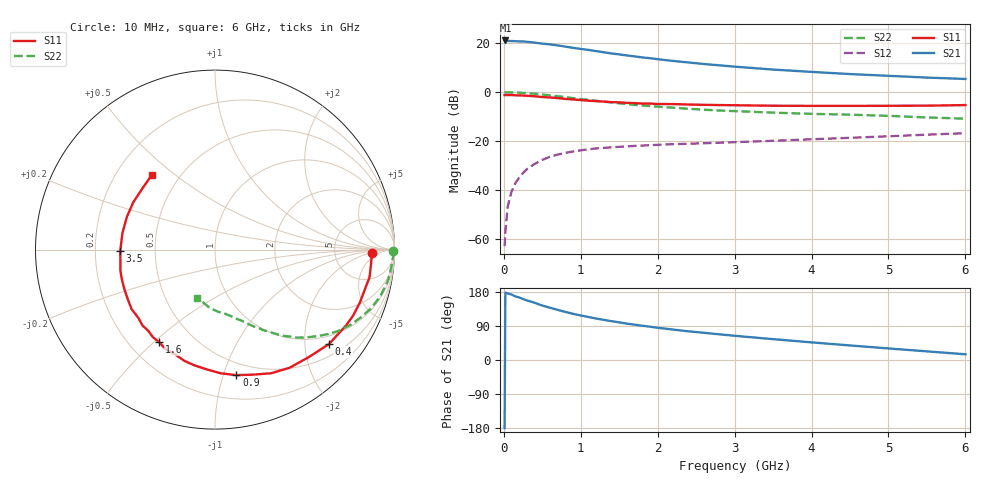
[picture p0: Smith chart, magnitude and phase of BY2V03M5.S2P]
! SIEMENS Small Signal Semiconductors
! BFY420
! Si NPN RF SIEGET Grounded Emitter Transistor in MICRO-X
! VCE = 2 V  IC = 3.5 mA
! Common Emitter S-Parameters:  October  1996
# GHz  S  MA  R  50
!  f  S11  S21  S12  S22
! GHz  MAG  ANG  MAG  ANG  MAG  ANG  MAG  ANG
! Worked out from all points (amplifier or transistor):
!   36 points, 10 MHz to 6 GHz, reference 50 ohm
!   highest |S21| = 21.2 dB at 20 MHz (marker M1)
!   |S21| within 3 dB of that: start of sweep to 893.2 MHz
!   unconditionally stable (mu >= 1): 3.446 GHz to end of sweep
!   at 250 MHz: K = 0.09, MSG = 27.0 dB, |S12| = -33.1 dB
!   at 1.4 GHz: K = 0.43, MSG = 19.2 dB, |S12| = -22.6 dB
!   at 6 GHz: K = 1.18, MAG = 8.5 dB, |S12| = -16.8 dB
!   S11 on the Smith chart (normalised r, x): 10 MHz: 15, -2; 400 MHz: 0.78, -2.57; 900 MHz: 0.39, -1.11; 1.6 GHz: 0.32, -0.52; 3.5 GHz: 0.31, -0.00; 6 GHz: 0.35, +0.41
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0.01  0.8737 -1.1  11.46 -179.9  0.0007 110.8  0.9941 -0.6
0.02  0.8738 -2.1  11.47 178.0  0.0014 84.1  0.994 -1.0
0.05  0.8731 -5.1  11.18 175.6  0.0045 91.6  0.9922 -2.6
0.1  0.8747 -10.1  11.17 172.8  0.0092 86.3  0.9871 -5.4
0.15  0.8639 -14.9  11.07 167.8  0.0137 80.0  0.9837 -8.1
0.2  0.8593 -20.2  10.99 165.0  0.0179 79.4  0.9771 -10.6
0.25  0.853 -25.5  10.95 160.9  0.0221 75.3  0.9659 -13.2
0.4  0.8249 -39.6  10.38 151.1  0.034 68.5  0.9282 -20.7
0.5  0.7952 -48.8  9.883 143.6  0.041 63.9  0.8947 -25.1
0.6  0.7785 -57.8  9.538 138.0  0.0475 59.9  0.8615 -29.3
0.7  0.7566 -65.6  9.087 132.3  0.0526 56.1  0.8264 -33.1
0.9  0.7095 -80.3  8.091 121.9  0.0611 49.3  0.7557 -39.4
1.1  0.6686 -94.1  7.346 113.4  0.0677 44.1  0.6944 -44.9
1.3  0.6429 -105.4  6.572 105.9  0.0724 40.3  0.6388 -49.3
1.6  0.6028 -121.1  5.652 95.9  0.0777 35.8  0.5704 -54.9
1.9  0.5849 -133.7  4.965 87.8  0.0822 32.7  0.5201 -59.4
2.2  0.5708 -144.6  4.361 80.3  0.0861 30.4  0.4812 -63.1
2.8  0.5448 -162.3  3.555 67.8  0.0921 27.8  0.4206 -69.8
3.5  0.5277 -179.4  2.907 55.0  0.101 26.2  0.3811 -76.5
4.5  0.5237 159.6  2.351 38.4  0.1161 23.2  0.3459 -87.4
5.5  0.5295 139.5  1.991 22.8  0.1348 19.4  0.3036 -101.9
6  0.5441 130.5  1.866 15.1  0.1444 16.9  0.287 -110.8
